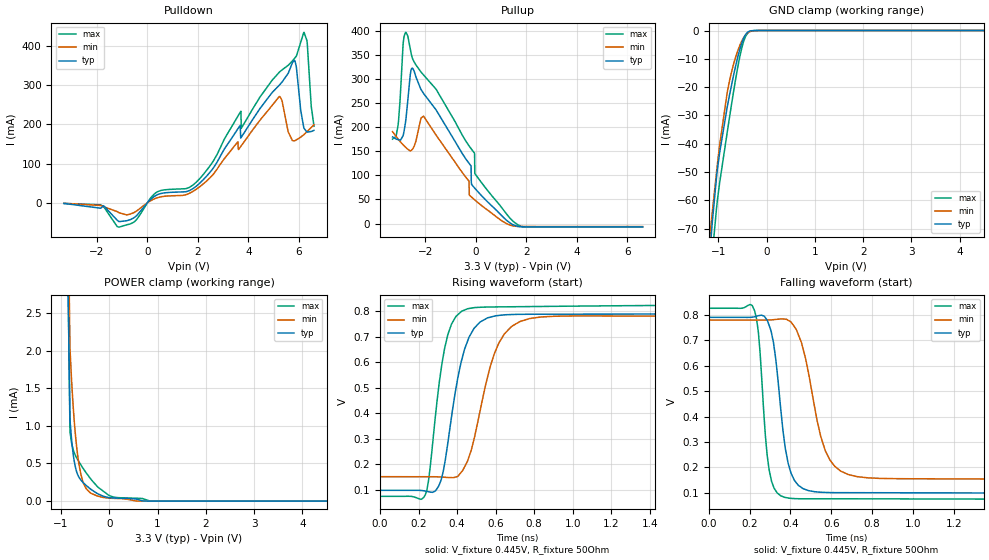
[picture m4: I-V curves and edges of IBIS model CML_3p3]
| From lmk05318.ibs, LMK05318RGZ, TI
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|   CML_3p3 Model
[Model]   CML_3p3
Model_type   3-state
Polarity   Non-Inverting
Vmeas = 0.445
Vref = 0.445
Cref = 2pF
Rref = 50
|   typ   min   max
C_comp   1.41794E-12   1.36037E-12   1.45091E-12
| Where nom  PVT is Nominal Process, 3.3V, 27C
|   Fast PVT is Strong Process,  3.45V, -40C
|   Slow PVT is Weak Process,   3.15V, 125C
[Voltage Range]   3.3   3.15   3.45
|Junction Temperature
[Temperature Range]   27   125   -40
[Pullup Reference]   3.3   3.15   3.45
[Pulldown Reference]   0   0   0
[Power Clamp Reference]   3.3   3.15   3.45
[GND Clamp Reference]   0   0   0
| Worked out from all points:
|   slope of the pulldown table from 0 to 0.495 V, typ, clamps not added: 21.6 ohm
|   slope of the pullup table from 0 to 0.495 V, typ, clamps not added: 18 ohm
|   GND clamp passes 1 mA (typ) near -0.41 V on its own axis
|   POWER clamp passes 1 mA (typ) near -0.80 V on its own axis
|   falling waveform, V_fixture 0.445V, R_fixture 50Ohm: 20-80 % time 60.3ps typ, 100ps min, 41.1ps max; typ from 0.791 V to 0.097 V
|   rising waveform, V_fixture 0.445V, R_fixture 50Ohm: 20-80 % time 96.6ps typ, 124ps min, 76.5ps max; typ from 0.097 V to 0.791 V
[Pulldown]
|   Voltage   I(typ)   I(min)   I(max)
-3.3V     -1.368mA   -1.115mA   -1.363mA
-1.845V   -13.51mA   -6.485mA   -4.855mA
-1.122V   -47.62mA   -24.89mA   -61.68mA
392.7mV   20.55mA    13.01mA    27.89mA
1.798V    35.9mA     28.87mA    44.92mA
3.699V    164.8mA    143.4mA    232.4mA
5.224V    299.1mA    270.5mA    332.1mA
5.828V    362.3mA    157.9mA    367.3mA
6.204V    189.6mA    173.8mA    433.8mA
6.323V    180.2mA    181.3mA    412.5mA
6.491V    181.5mA    191.8mA    245.8mA
6.6V      184.5mA    198.7mA    194.9mA
[GND Clamp]
|   Voltage   I(typ)   I(min)   I(max)
-3.3V     -1.225A    -1.029A    -1.515A
-1.181V   -80.15mA   -73.74mA   -92.54mA
-1.132V   -69.26mA   -65.41mA   -80.58mA
-1.122V   -67.19mA   -63.77mA   -78.45mA
-1.033V   -51.11mA   -49.44mA   -62.14mA
-973.5mV  -43.33mA   -40.6mA    -53.92mA
-815.1mV  -26.99mA   -21.86mA   -35.94mA
-765.6mV  -22.62mA   -17.58mA   -30.43mA
-528mV    -5.185mA   -4.26mA    -7.227mA
-438.9mV  -1.534mA   -1.654mA   -2.27mA
-349.8mV  -210.4uA   -427.7uA   -364.9uA
6.6V      0A         0A         0A
[Pullup]
|   Voltage   I(typ)   I(min)   I(max)
-3.3V     180mA      190.9mA    175.4mA
-3.082V   174.3mA    175.9mA    203.6mA
-2.884V   182.3mA    163.8mA    370.6mA
-2.765V   219.1mA    157.7mA    397.2mA
-2.498V   322.1mA    155.4mA    341.5mA
-2.072V   270.4mA    223.2mA    308.8mA
-270.6mV  125mA      87.9mA     161.4mA
-260.7mV  124.3mA    59.16mA    160.7mA
-52.8mV   73.94mA    49.39mA    146mA
-42.9mV   73.35mA    48.94mA    104mA
1.511V    -3.524mA   -5.364mA   2.928mA
6.6V      -6.964mA   -6.294mA   -7.577mA
[POWER Clamp]
|   Voltage   I(typ)   I(min)   I(max)
-3.3V     2.746A     3.266A     2.249A
-1.488V   31.11mA    34.76mA    35.04mA
-815.1mV  1.082mA    2.027mA    921.9uA
-775.5mV  776.3uA    1.532mA    752.1uA
-726mV    528.1uA    1.059mA    641.3uA
-627mV    314.2uA    482.9uA    520.1uA
-557.7mV  256.3uA    280uA      449.6uA
-478.5mV  207.7uA    164.7uA    374.7uA
-260.7mV  105.7uA    70.86uA    202.7uA
75.9mV    41.45uA    37.03uA    56.03uA
897.6mV   0A         127.3nA    190.5nA
6.6V      0A         0A         0A
[Ramp]
R_load = 50
|   typ   min   max
dV/dt_r   0.416201/9.66196e-11   0.377767/1.24361e-10   0.451806/7.65254e-11
dV/dt_f   0.416388/6.02564e-11   0.377548/1.00289e-10   0.451855/4.10797e-11
[Falling Waveform]
V_fixture = 0.445V
V_fixture_min = 0.466V
V_fixture_max = 0.452V
R_fixture = 50Ohm
C_fixture = 0F
|   Time   V(typ)   V(min)   V(max)
0s        791.1mV    780.6mV    826.9mV
225.1ps   793.5mV    780.5mV    816.6mV
243.2ps   797.6mV    780.4mV    732.9mV
296.2ps   758.9mV    780.8mV    188.3mV
328.6ps   625.8mV    782.9mV    107.3mV
371.1ps   299mV      784.3mV    81.79mV
438.4ps   129.3mV    723.8mV    76.22mV
571ps     101mV      265.3mV    75.97mV
683.2ps   99.97mV    171.5mV    75.96mV
2.5ns     97.16mV    151.4mV    73.81mV
[Rising Waveform]
V_fixture = 0.445V
V_fixture_min = 0.466V
V_fixture_max = 0.452V
R_fixture = 50Ohm
C_fixture = 0F
|   Time   V(typ)   V(min)   V(max)
0s        97.33mV    151mV      73.77mV
234.5ps   94.7mV     150.8mV    78.73mV
251.7ps   91.98mV    150.9mV    134.8mV
305.1ps   115mV      150.2mV    505.1mV
328.6ps   172.9mV    149.1mV    625.5mV
371.1ps   386mV      147.3mV    750mV
455.2ps   684.7mV    214.2mV    810.3mV
592.9ps   781.1mV    633mV      817.2mV
726.1ps   788.2mV    760mV      818.2mV
2.5ns     791mV      780.6mV    826.8mV
